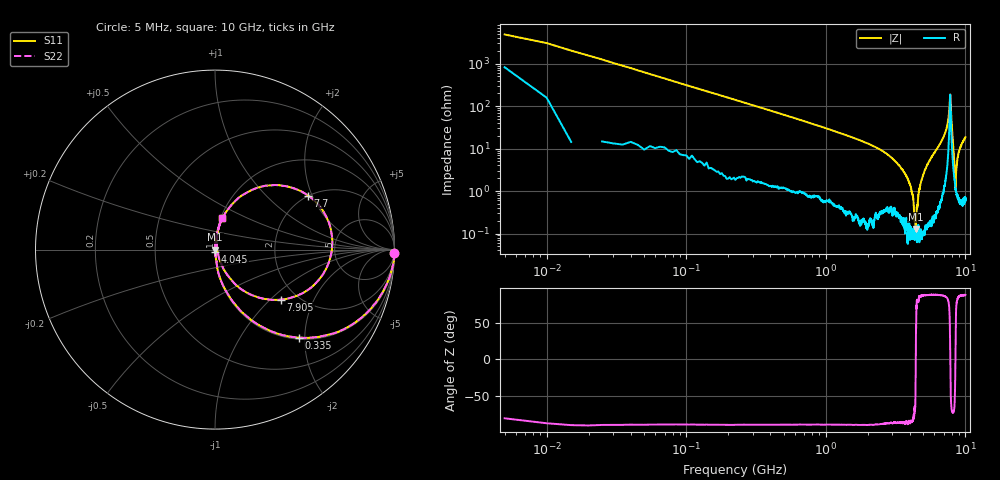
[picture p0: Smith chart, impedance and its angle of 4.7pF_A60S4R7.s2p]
! Amotech Co.,Ltd.
! http://www.amotech.co.kr/
! Part Number: A60S4R7
! These Parameters are Measured in Series Mode Connection
! Operation Temp=25[degC], DC Bias Voltage=0[V]
! Freq. Start=5[MHz] Stop=10[GHz], 2000[Steps]
! Date: Monday, July 13, 2020, 01:55:11
# GHZ S RI R 50.000000
!Freq.(Hz) S11(Real) S11(Imag) S21(Real) S21(Imag) S12(Real) S12(Imag) S22(Real) S22(Imag)
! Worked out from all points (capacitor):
!   2000 points, 5 MHz to 10 GHz, reference 50 ohm
!   read as one part in series: C = 5.08 pF near 55 MHz
!   lowest |Z| = 127 mohm at 4.395 GHz (marker M1)
!   series resonance near 4.411 GHz, so ESL is about 260 pH
!   S11 on the Smith chart (normalised r, x): 5 MHz: 17, -96; 335 MHz: 1.03, -1.88; 4.045 GHz: 1.00, -0.03; 7.7 GHz: 1.98, +1.86; 7.905 GHz: 1.65, -1.17; 10 GHz: 1.01, +0.37
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0.005  0.9961 -0.02  0.00385 0.02  0.00385 0.02  0.9961 -0.02
0.11  0.8842 -0.3082  0.1158 0.3082  0.1158 0.3082  0.8842 -0.3082
0.335  0.4697 -0.4905  0.5303 0.4905  0.5303 0.4905  0.4697 -0.4905
0.765  0.1449 -0.3424  0.8551 0.3424  0.8551 0.3424  0.1449 -0.3424
1.675  0.0294 -0.1611  0.9706 0.1611  0.9706 0.1611  0.0294 -0.1611
3.34  0.00424 -0.0398  0.9958 0.0398  0.9958 0.0398  0.00424 -0.0398
4.045  0.0011 -0.0131  0.9989 0.0131  0.9989 0.0131  0.0011 -0.0131
4.22  0.000974 -0.00738  0.999 0.00738  0.999 0.00738  0.000974 -0.00738
4.395  0.00107 -0.000673  0.9989 0.000673  0.9989 0.000673  0.00107 -0.000673
4.645  0.000837 0.00943  0.9992 -0.00943  0.9992 -0.00943  0.000837 0.00943
5.005  0.00157 0.0252  0.9984 -0.0252  0.9984 -0.0252  0.00157 0.0252
6.67  0.0247 0.1357  0.9753 -0.1357  0.9753 -0.1357  0.0247 0.1357
7.41  0.1319 0.2883  0.8681 -0.2883  0.8681 -0.2883  0.1319 0.2883
7.7  0.5173 0.3014  0.4827 -0.3014  0.4827 -0.3014  0.5173 0.3014
7.79  0.6515 0.00522  0.3485 -0.00522  0.3485 -0.00522  0.6515 0.00522
7.905  0.3683 -0.2783  0.6317 0.2783  0.6317 0.2783  0.3683 -0.2783
8.06  0.1084 -0.1886  0.8916 0.1886  0.8916 0.1886  0.1084 -0.1886
8.335  0.0206 -0.0418  0.9794 0.0418  0.9794 0.0418  0.0206 -0.0418
8.49  0.0109 0.00292  0.9891 -0.00292  0.9891 -0.00292  0.0109 0.00292
8.64  0.0099 0.0356  0.9901 -0.0356  0.9901 -0.0356  0.0099 0.0356
8.94  0.0124 0.0781  0.9876 -0.0781  0.9876 -0.0781  0.0124 0.0781
10  0.0392 0.1781  0.9608 -0.1781  0.9608 -0.1781  0.0392 0.1781
